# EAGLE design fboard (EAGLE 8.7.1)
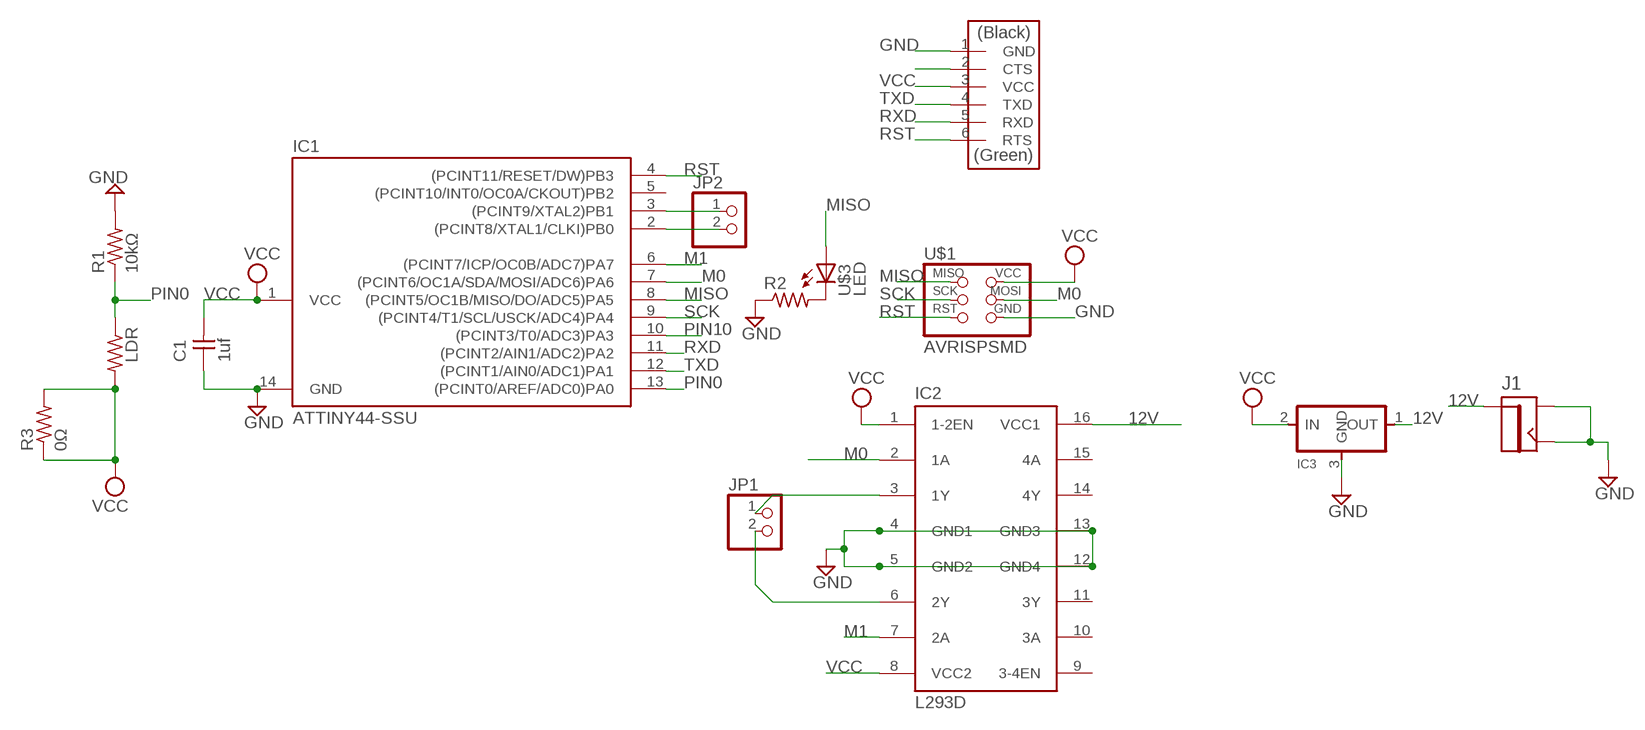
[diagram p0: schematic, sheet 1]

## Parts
C1  1uf  CAP-UNPOLARIZEDFAB  [C1206FAB]
IC1  ATTINY44-SSU  [SOIC14]
IC2  L293D  [DIL16]
IC3  REGULATORSOT23  [SOT23]
J1  JACK.65MM  [JACK_.65MM]
JP1  PINHD-1X2  [1X02]
JP2  PINHD-1X2  [1X02]
LDR  R-US_0204/5  [0204/5]
R1  10kΩ  RES-US1206FAB  [R1206FAB]
R2  RES-US1206FAB  [R1206FAB]
R3  0Ω  RES-US1206FAB  [R1206FAB]
U$1  AVRISPSMD  [2X03SMD]
U$2  FTDI-SMD-HEADER  [1X06SMD]
U$3  LED  [LED1206]

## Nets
12V: IC2.16(VCC1) IC3.1(OUT) J1.PIN
GND: C1.1 IC1.14(GND) IC2.4(GND1) IC2.5(GND2) IC2.12(GND4) IC2.13(GND3) IC3.3(GND) J1.CONTACT(SHUNT) J1.SHUNT(CONTACT) R1.2 R2.1 U$1.6(GND) U$2.1(GND)
M0: IC1.7((PCINT6/OC1A/SDA/MOSI/ADC6)PA6) IC2.2(1A) U$1.4(MOSI)
M1: IC1.6((PCINT7/ICP/OC0B/ADC7)PA7) IC2.7(2A)
MISO: IC1.8((PCINT5/OC1B/MISO/DO/ADC5)PA5) U$1.1(MISO) U$3.1(A)
N$1: IC1.3((PCINT9/XTAL2)PB1) JP2.1
N$3: IC1.2((PCINT8/XTAL1/CLKI)PB0) JP2.2
N$4: U$2.2(CTS)
N$6: R2.2 U$3.2(C)
N$7: IC2.3(1Y) JP1.1
N$8: IC2.6(2Y) JP1.2
PIN0: IC1.13((PCINT0/AREF/ADC0)PA0) LDR.1 R1.1
PIN10: IC1.10((PCINT3/T0/ADC3)PA3)
RST: IC1.4((PCINT11/RESET/DW)PB3) U$1.5(RST) U$2.6(RTS)
RXD: IC1.11((PCINT2/AIN1/ADC2)PA2) U$2.5(RXD)
SCK: IC1.9((PCINT4/T1/SCL/USCK/ADC4)PA4) U$1.3(SCK)
TXD: IC1.12((PCINT1/AIN0/ADC1)PA1) U$2.4(TXD)
VCC: C1.2 IC1.1(VCC) IC2.1(1-2EN) IC2.8(VCC2) IC3.2(IN) LDR.2 R3.1 R3.2 U$1.2(VCC) U$2.3(VCC)
Unconnected: IC1.5((PCINT10/INT0/OC0A/CKOUT)PB2) IC2.9(3-4EN) IC2.10(3A) IC2.11(3Y) IC2.14(4Y) IC2.15(4A)

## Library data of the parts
C1 = fab (1):CAP-UNPOLARIZED
IC1 = fab (1):ATTINY44
IC2 = st-microelectronics:L293D: PUSH-PULL 4 CHANNEL DRIVER; MPN: L293D; OC_FARNELL: 9589619; OC_NEWARK: 56P8249
IC3 = fab (1):REGULATOR
J1 = fab (1):JACK
JP1 JP2 = pinhead:PINHD-1X2: PIN HEADER
LDR = resistor:R-US_: RESISTOR, American symbol
R1-R3 = fab (1):RES-US: Resistor (US Symbol)
U$1 = fab (1):AVRISP
U$2 = fab (1):FTDI-SMD-HEADER
U$3 = fab (1):LED: LED

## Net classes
0 fab: width 0.35 mm, drill 0.4 mm, clearance 0.315 mm

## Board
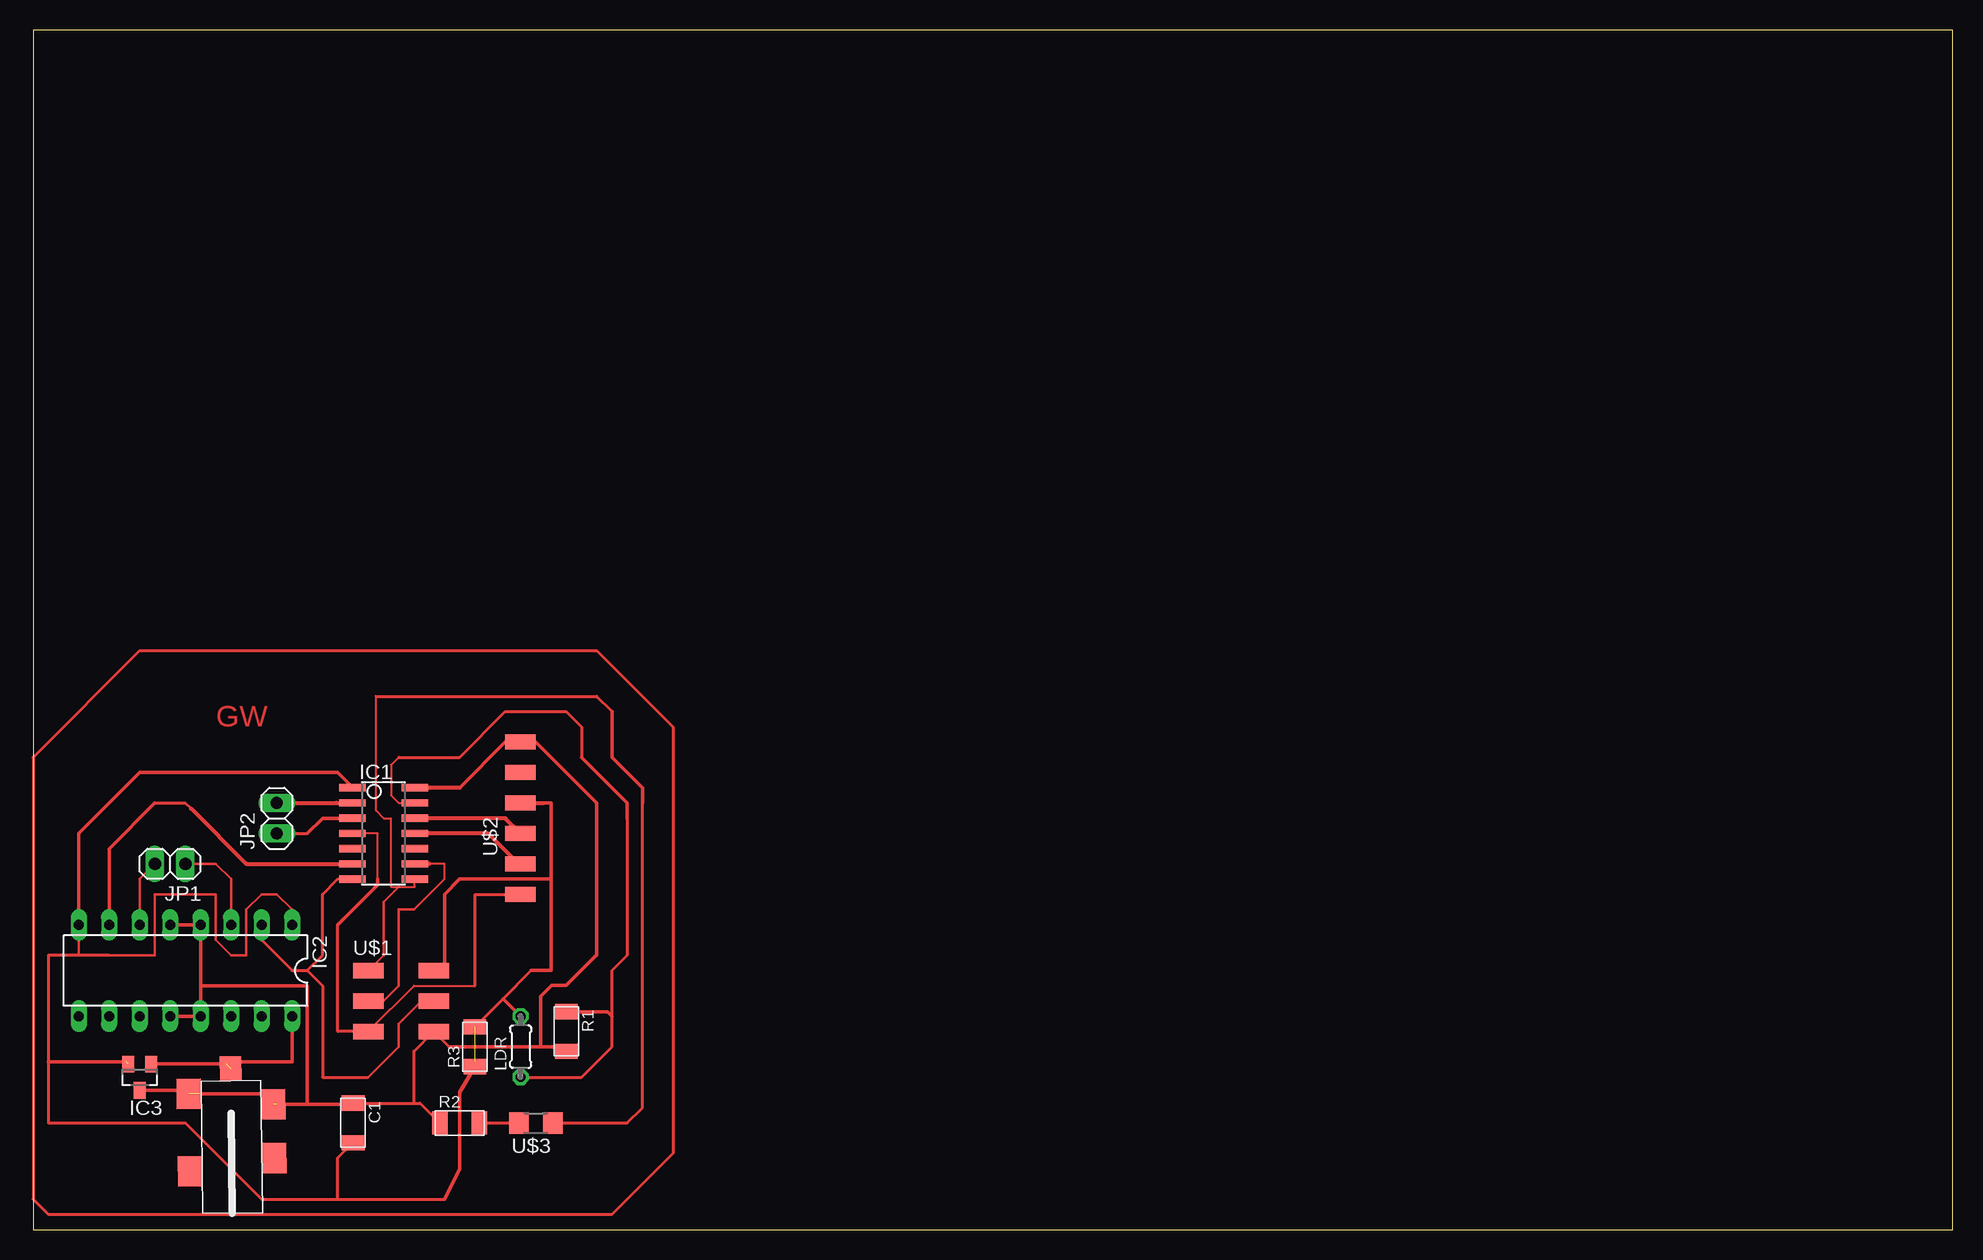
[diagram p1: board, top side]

Size 160 x 100 mm. Coordinates in mm from the lower left corner, seen from the top.
Outline: 0,0 160,0 160,100 0,100 0,0
Copper layers (1*16): Top 0.035mm / dielectric 1.5mm / Bottom 0.035mm
Design rules "fab": minimum track width 0.3mm, minimum drill 32mil, track to track 0.315mm, track to pad 0.315mm, pad to pad 0.315mm, via to via 0.315mm, smd to smd 0.315mm, copper to edge 40mil, drill to drill 16mil, minimum pad ring 10mil, minimum via ring 8mil, stop-mask expansion 4mil, vias tented up to drill 0mil, thermal gap 10mil

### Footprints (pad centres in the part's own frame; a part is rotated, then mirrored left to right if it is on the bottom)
C1206FAB = smd 1.27 x 1.905: 1 -1.651,0; 2 1.651,0
SOIC14 = smd 0.61 x 2.21: 1 -3.81,-2.603; 2 -2.54,-2.603; 3 -1.27,-2.603; 4 0,-2.603; 5 1.27,-2.603; 6 2.54,-2.603; 7 3.81,-2.603; 8 3.81,2.603; 9 2.54,2.603; 10 1.27,2.603; 11 0,2.603; 12 -1.27,2.603; 13 -2.54,2.603; 14 -3.81,2.603
DIL16 = drill 0.813 long: 1 -8.89,-3.81; 2 -6.35,-3.81; 3 -3.81,-3.81; 4 -1.27,-3.81; 5 1.27,-3.81; 6 3.81,-3.81; 7 6.35,-3.81; 8 8.89,-3.81; 9 8.89,3.81; 10 6.35,3.81; 11 3.81,3.81; 12 1.27,3.81; 13 -1.27,3.81; 14 -3.81,3.81; 15 -6.35,3.81; 16 -8.89,3.81
SOT23 = smd 1 x 1.4: 1 -0.95,-1.1; 2 0.95,-1.1; 3 0,1.1
JACK_.65MM = smd 2.032 x 2.54: CONTACT 3.578,4.026; SHIELD -3.45,-1.448; SHIELD1 3.578,-0.447; SHUNT -3.45,5.005 | smd 1.778 x 2.032: PIN 0.064,7.071
1X02 = drill 1.016 long: 1 -1.27,0; 2 1.27,0
0204/5 = drill 0.813 octagon: 1 -2.54,0; 2 2.54,0
R1206FAB = smd 1.27 x 1.905: 1 -1.651,0; 2 1.651,0
2X03SMD = smd 2.54 x 1.27: 1 -2.54,2.54; 2 2.92,2.54; 3 -2.54,0; 4 2.92,0; 5 -2.54,-2.54; 6 2.92,-2.54
1X06SMD = smd 2.54 x 1.27: 1 0,6.35; 2 0,3.81; 3 0,1.27; 4 0,-1.27; 5 0,-3.81; 6 0,-6.35
LED1206 = smd 1.6 x 1.803: 1 -1.422,0; 2 1.422,0

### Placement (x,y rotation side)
C1  26.67,8.89 270 top
IC1  29.21,33.02 270 top
IC2  12.7,21.59 180 top
IC3  8.89,12.7 180 top
J1  16.51,6.35 0.8 top
JP1  11.43,30.48 180 top
JP2  20.32,34.29 90 top
LDR  40.64,15.24 90 top
R1  44.45,16.51 270 top
R2  35.56,8.89 0 top
R3  36.83,15.24 90 top
U$1  30.48,19.05 0 top
U$2  40.64,34.29 0 top
U$3  41.91,8.89 180 top

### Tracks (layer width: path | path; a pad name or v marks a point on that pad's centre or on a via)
12V  (1 unrouted)
  Top 0.305: IC3.1 16.1,13.8 | 21.59,16.51 IC2.16 21.59,13.97 17.02,13.97 J1.PIN
GND  (2 unrouted)
  Top 0.152: 13.97,11.43 13.85,11.31
  Top 0.254: 20.32,10.43 19.82,10.93 | C1.1 31.75,10.54 | 31.75,10.54 32.26,10.54 R2.1 | 31.75,10.54 31.75,14.86 U$1.6 34.67,15.24
  Top 0.305: 42.29,15.24 42.29,19.43 43.23,20.37 44.45,20.37 46.94,22.86 46.99,22.86 46.99,35.56 41.91,40.64 U$2.1 39.37,40.64 35.56,36.83 | 19.82,10.93 19.44,11.31 J1.SHUNT 12.7,11.6 IC3.3 | J1.CONTACT 22.86,10.43 | 22.86,10.43 26.55,10.43 C1.1 | 13.97,20.32 IC2.4 IC2.5 | 13.97,20.32 IC2.13 IC2.12 | 13.97,20.32 22.86,20.32 22.86,10.43 | 34.67,15.24 42.29,15.24 | 42.29,15.24 44.07,15.24 R1.2
  Top 0.35: 35.56,36.83 IC1.14 | 40.48,40.64 U$2.1 40.8,40.64
M0
  Top 0.152: IC1.7 25.4,29.21
  Top 0.203: U$1.4 32.38,19.05 30.8,17.46 30.48,17.14 30.48,15.24 27.94,12.7
  Top 0.254: 25.4,29.21 24.13,27.94 24.13,22.86 22.86,21.59 | IC2.2 19.05,24.13 21.59,21.59 22.86,21.59 | 22.86,21.59 24.13,20.32 24.13,12.7 27.94,12.7
M1
  Top 0.254: 10.16,35.56 12.7,35.56 13.18,35.08
  Top 0.305: IC2.7 6.35,31.75 10.16,35.56
  Top 0.35: IC1.6 17.78,30.48 13.18,35.08
MISO
  Top 0.152: 28.58,44.45 28.58,34.92 29.21,34.29 29.84,34.29 29.84,28.57 30.48,28.57 31.81,28.57 IC1.8
  Top 0.203: 30.48,28.57 29.21,27.3 29.21,22.86 U$1.1
  Top 0.254: 28.58,44.45 46.99,44.45 48.26,43.18 | U$3.1 49.53,8.89 50.8,10.16 50.8,35.56
  Top 0.305: 50.8,35.56 50.8,36.83 48.26,39.37 48.26,43.18
N$1
  Top 0.254: JP2.1 22.86,33.02
  Top 0.305: 22.86,33.02 24.13,34.29 26.56,34.29 26.6,34.25
  Top 0.35: 26.6,34.25 IC1.3 | 20.61,33.25 JP2.1
N$2
  Top 0.254: 8.89,48.26 46.99,48.26 53.34,41.91 53.34,6.35 48.26,1.27 1.27,1.27 0,2.54 0,39.37 8.89,48.26
N$3
  Top 0.35: IC1.2 25.4,35.56 25.27,35.58 20.61,35.58 JP2.2
N$6
  Top 0.254: 36.83,8.51 R2.2 U$3.2
N$7
  Top 0.203: JP1.1 15.24,30.48 16.51,29.21 IC2.3
  Top 0.35: 12.97,30.26 JP1.1
N$8
  Top 0.203: IC2.6 8.89,29.21 JP1.2
  Top 0.35: 8.98,25.6 IC2.6 | 9.97,30.26 JP1.2
PIN0
  Top 0.152: IC1.13 30.48,35.56 29.84,36.2 29.84,38.73 30.48,39.37
  Top 0.254: 45.72,39.37 45.72,41.91 44.45,43.18 39.37,43.18 35.56,39.37 30.48,39.37 | 49.53,34.29 49.53,22.86 48.26,21.59 48.26,17.78 48.26,15.24 45.72,12.7 LDR.1 | 44.83,18.16 R1.1
  Top 0.305: R1.1 47.88,18.16 48.26,17.78 | 45.72,39.37 49.53,35.56 49.53,34.29
RST
  Top 0.152: IC1.4 28.74,33.02 28.74,29.21 | U$1.5 31.75,20.32 36.81,20.32 36.82,20.33
  Top 0.254: U$1.5 25.4,16.51 25.4,25.4 | 39.57,27.93 36.82,27.93 36.82,20.33 36.83,20.32
  Top 0.305: 25.4,25.4 28.74,28.74 28.74,29.21
  Top 0.35: 39.57,27.93 U$2.6 | 27.3,16.51 U$1.5
RXD
  Top 0.35: IC1.11 37.94,33.02 40.48,30.48 U$2.5
SCK
  Top 0.152: 33.02,30.48 34.29,30.48 34.29,29.21 31.75,26.67
  Top 0.203: U$1.3 29.21,19.05 30.48,20.32 30.48,26.67 31.75,26.67
  Top 0.35: IC1.9 33.02,30.48 | U$1.3 28.57,19.05
TXD
  Top 0.35: IC1.12 39.37,34.29 U$2.4
VCC  (2 unrouted)
  Top 0.203: IC2.1 21.59,26.67 20.32,27.94 19.05,27.94 17.78,26.67 17.78,22.86 16.51,22.86 15.24,24.13 15.24,27.94 10.16,27.94 10.16,22.86 6.35,22.86 | IC2.8 3.81,22.86
  Top 0.254: 6.35,22.86 3.81,22.86 1.27,22.86 1.27,13.97 1.27,8.89 12.7,8.89 19.05,2.54 25.4,2.54 | 25.4,2.54 25.4,5.97 C1.2 | 25.4,2.54 34.29,2.54 | 36.83,13.97 R3.1 | R3.2 39.18,19.24 41.53,21.59
  Top 0.305: IC2.8 3.81,33.02 8.89,38.1 25.4,38.1 26.61,36.89 IC1.1 | 42.55,35.56 43.18,35.56 43.18,29.21 | 43.18,29.21 43.18,21.59 41.53,21.59 | 34.29,2.54 35.56,5.08 35.56,11.43 R3.1 | LDR.2 39.18,19.24 | 1.27,13.97 7.77,13.97 | 34.29,22.23 34.29,27.94 35.56,29.21 43.18,29.21
  Top 0.35: 3.97,25.4 IC2.8 3.99,25.6 | IC1.1 26.6,36.91 | 40.9,35.24 U$2.3 42.55,35.56 | 34.29,22.23 33.66,21.59 U$1.2

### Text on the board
Top: GW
